(* Logix 5000 AddOnInstructionDefinition export; software revision 16.04 *)

ADD_ON_INSTRUCTION AOI_ICX35   (* revision 1.8 *)
// Add-On Instruction for ICX35 Industrial Cellular Gateway
// Revision note:
// 1.8    2018/06/14.
// This Revision is compatible with ICX35 firmware version 1.4 and later.
VAR_IN_OUT
   ICX35 : ICX35_ModuleDef; {required}
   ICX35_MSG_GET_STATUS : MESSAGE; {required}
   ICX35_MSG_READ_SMS : MESSAGE; {required}
   ICX35_MSG_RESET_STATUS : MESSAGE; {required}
   ICX35_MSG_WRITE_SMS : MESSAGE; {required}
   ICX35_MSG_CLEAR_SMS : MESSAGE; {required}
   ICX35_MSG_REBOOT : MESSAGE; {required}
END_VAR

ROUTINE Logic   (* ladder *)
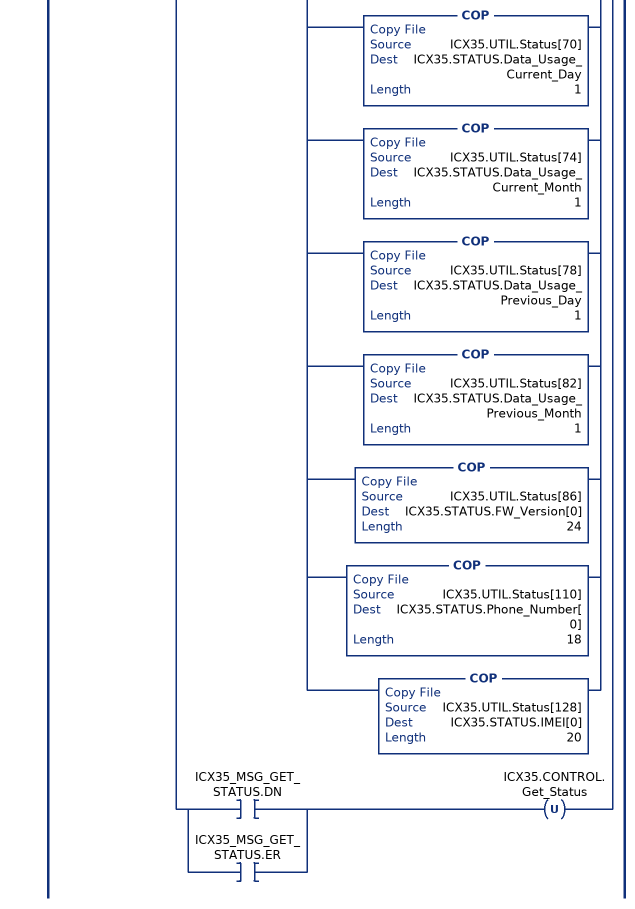
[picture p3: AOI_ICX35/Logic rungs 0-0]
   0: XIC(ICX35.CONTROL.Get_Status)[MSG(ICX35_MSG_GET_STATUS) ,XIC(ICX35_MSG_GET_STATUS.DN) [COP(ICX35.UTIL.Status[0],ICX35.STATUS.RSSI,4) ,COP(ICX35.UTIL.Status[4],ICX35.STATUS.MAC_Address[0],6) ,MVM(0,65280,ICX35.STATUS.WAN_IP[0]) ,MVM(ICX35.UTIL.Status[10],255,ICX35.STATUS.WAN_IP[0]) ,MVM(0,65280,ICX35.STATUS.WAN_IP[1]) ,MVM(ICX35.UTIL.Status[11],255,ICX35.STATUS.WAN_IP[1]) ,MVM(0,65280,ICX35.STATUS.WAN_IP[2]) ,MVM(ICX35.UTIL.Status[12],255,ICX35.STATUS.WAN_IP[2]) ,MVM(0,65280,ICX35.STATUS.WAN_IP[3]) ,MVM(ICX35.UTIL.Status[13],255,ICX35.STATUS.WAN_IP[3]) ,COP(ICX35.UTIL.Status[14],ICX35.STATUS.Cell_Net_Disconnects,1) ,COP(ICX35.UTIL.Status[18],ICX35.STATUS.LAN_KBytes_Sent,1) ,COP(ICX35.UTIL.Status[22],ICX35.STATUS.LAN_KBytes_Received,1) ,COP(ICX35.UTIL.Status[26],ICX35.STATUS.WAN_KBytes_Sent,1) ,COP(ICX35.UTIL.Status[30],ICX35.STATUS.WAN_KBytes_Received,1) ,COP(ICX35.UTIL.Status[34],ICX35.STATUS.SMS_MSGs_Sent,1) ,COP(ICX35.UTIL.Status[38],ICX35.STATUS.SMS_MSGs_Received,1) ,COP(ICX35.UTIL.Status[42],ICX35.STATUS.SMS_MSGs_Rx_Free_Buffer_Counter,1) ,COP(ICX35.UTIL.Status[46],ICX35.STATUS.PowerOnTime_Year,1) ,COP(ICX35.UTIL.Status[48],ICX35.STATUS.PowerOnTime_Month,1) ,COP(ICX35.UTIL.Status[50],ICX35.STATUS.PowerOnTime_Day,1) ,COP(ICX35.UTIL.Status[52],ICX35.STATUS.PowerOnTime_Hour,1) ,COP(ICX35.UTIL.Status[54],ICX35.STATUS.PowerOnTime_Minute,1) ,COP(ICX35.UTIL.Status[56],ICX35.STATUS.PowerOnTime_Second,1) ,COP(ICX35.UTIL.Status[58],ICX35.STATUS.Link_Time_Days,1) ,COP(ICX35.UTIL.Status[62],ICX35.STATUS.Link_Time_Hours,1) ,COP(ICX35.UTIL.Status[66],ICX35.STATUS.Link_Time_Minutes,1) ,COP(ICX35.UTIL.Status[68],ICX35.STATUS.Link_Time_Seconds,1) ,COP(ICX35.UTIL.Status[70],ICX35.STATUS.Data_Usage_Current_Day,1) ,COP(ICX35.UTIL.Status[74],ICX35.STATUS.Data_Usage_Current_Month,1) ,COP(ICX35.UTIL.Status[78],ICX35.STATUS.Data_Usage_Previous_Day,1) ,COP(ICX35.UTIL.Status[82],ICX35.STATUS.Data_Usage_Previous_Month,1) ,COP(ICX35.UTIL.Status[86],ICX35.STATUS.FW_Version[0],24) ,COP(ICX35.UTIL.Status[110],ICX35.STATUS.Phone_Number[0],18) ,COP(ICX35.UTIL.Status[128],ICX35.STATUS.IMEI[0],20) ] ,[XIC(ICX35_MSG_GET_STATUS.DN) ,XIC(ICX35_MSG_GET_STATUS.ER) ] OTU(ICX35.CONTROL.Get_Status) ];
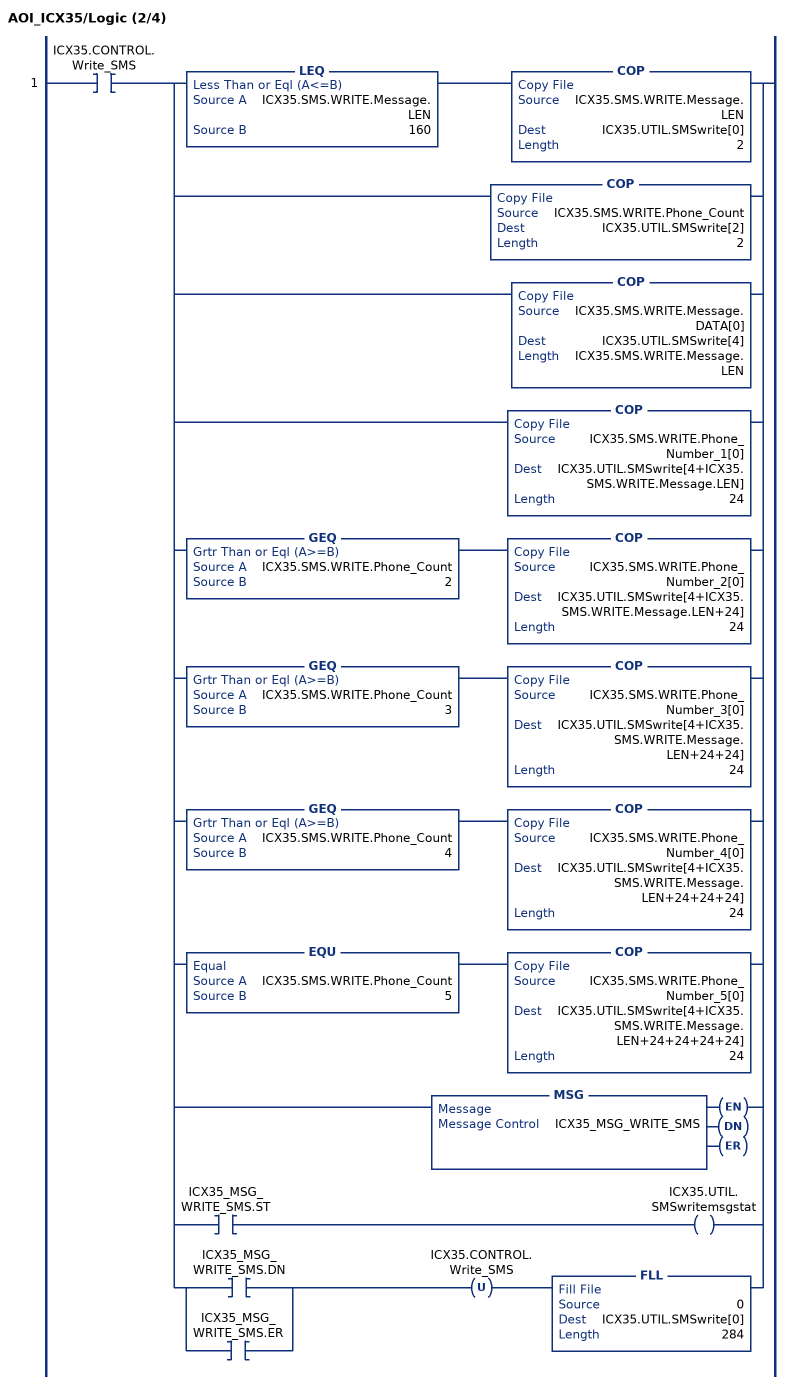
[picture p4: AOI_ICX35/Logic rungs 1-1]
   1: XIC(ICX35.CONTROL.Write_SMS)[LEQ(ICX35.SMS.WRITE.Message.LEN,160) COP(ICX35.SMS.WRITE.Message.LEN,ICX35.UTIL.SMSwrite[0],2) ,COP(ICX35.SMS.WRITE.Phone_Count,ICX35.UTIL.SMSwrite[2],2) ,COP(ICX35.SMS.WRITE.Message.DATA[0],ICX35.UTIL.SMSwrite[4],ICX35.SMS.WRITE.Message.LEN) ,COP(ICX35.SMS.WRITE.Phone_Number_1[0],ICX35.UTIL.SMSwrite[4+ICX35.SMS.WRITE.Message.LEN],24) ,GEQ(ICX35.SMS.WRITE.Phone_Count,2) COP(ICX35.SMS.WRITE.Phone_Number_2[0],ICX35.UTIL.SMSwrite[4+ICX35.SMS.WRITE.Message.LEN+24],24) ,GEQ(ICX35.SMS.WRITE.Phone_Count,3) COP(ICX35.SMS.WRITE.Phone_Number_3[0],ICX35.UTIL.SMSwrite[4+ICX35.SMS.WRITE.Message.LEN+24+24],24) ,GEQ(ICX35.SMS.WRITE.Phone_Count,4) COP(ICX35.SMS.WRITE.Phone_Number_4[0],ICX35.UTIL.SMSwrite[4+ICX35.SMS.WRITE.Message.LEN+24+24+24],24) ,EQU(ICX35.SMS.WRITE.Phone_Count,5) COP(ICX35.SMS.WRITE.Phone_Number_5[0],ICX35.UTIL.SMSwrite[4+ICX35.SMS.WRITE.Message.LEN+24+24+24+24],24) ,MSG(ICX35_MSG_WRITE_SMS) ,XIC(ICX35_MSG_WRITE_SMS.ST) OTE(ICX35.UTIL.SMSwritemsgstat) ,[XIC(ICX35_MSG_WRITE_SMS.DN) ,XIC(ICX35_MSG_WRITE_SMS.ER) ] OTU(ICX35.CONTROL.Write_SMS) FLL(0,ICX35.UTIL.SMSwrite[0],284) ];
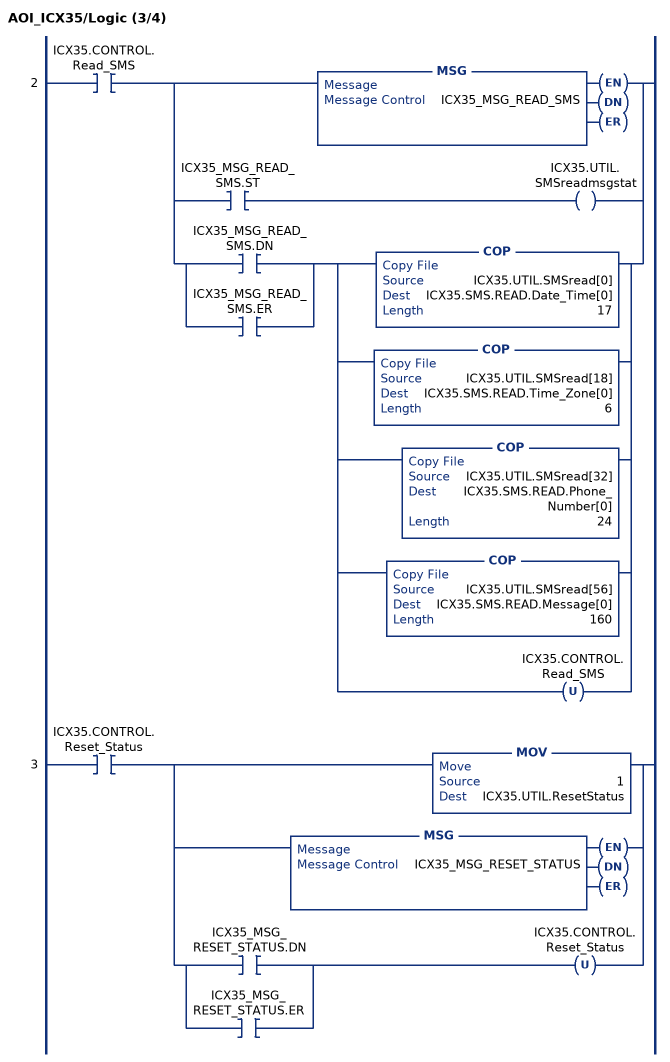
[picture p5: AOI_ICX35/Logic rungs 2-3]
   2: XIC(ICX35.CONTROL.Read_SMS)[MSG(ICX35_MSG_READ_SMS) ,XIC(ICX35_MSG_READ_SMS.ST) OTE(ICX35.UTIL.SMSreadmsgstat) ,[XIC(ICX35_MSG_READ_SMS.DN) ,XIC(ICX35_MSG_READ_SMS.ER) ] [COP(ICX35.UTIL.SMSread[0],ICX35.SMS.READ.Date_Time[0],17) ,COP(ICX35.UTIL.SMSread[18],ICX35.SMS.READ.Time_Zone[0],6) ,COP(ICX35.UTIL.SMSread[32],ICX35.SMS.READ.Phone_Number[0],24) ,COP(ICX35.UTIL.SMSread[56],ICX35.SMS.READ.Message[0],160) ,OTU(ICX35.CONTROL.Read_SMS) ] ];
   3: XIC(ICX35.CONTROL.Reset_Status)[MOV(1,ICX35.UTIL.ResetStatus) ,MSG(ICX35_MSG_RESET_STATUS) ,[XIC(ICX35_MSG_RESET_STATUS.DN) ,XIC(ICX35_MSG_RESET_STATUS.ER) ] OTU(ICX35.CONTROL.Reset_Status) ];
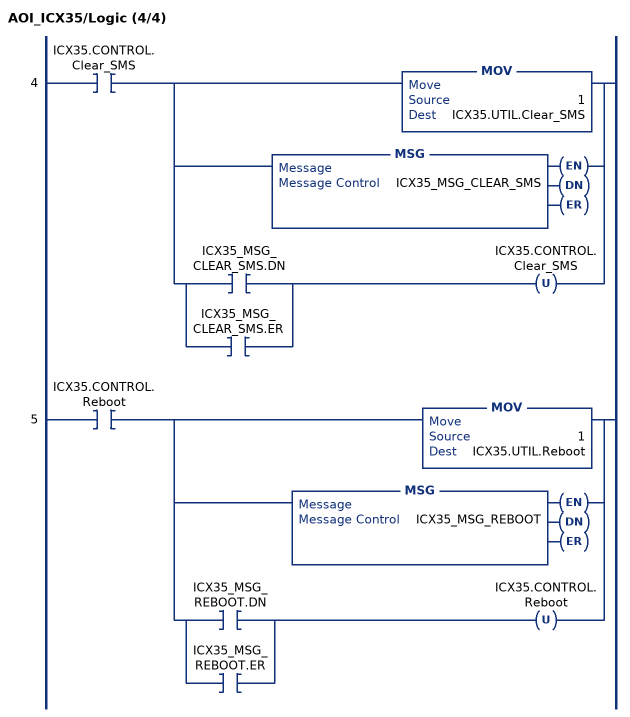
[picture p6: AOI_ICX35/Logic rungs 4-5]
   4: XIC(ICX35.CONTROL.Clear_SMS)[MOV(1,ICX35.UTIL.Clear_SMS) ,MSG(ICX35_MSG_CLEAR_SMS) ,[XIC(ICX35_MSG_CLEAR_SMS.DN) ,XIC(ICX35_MSG_CLEAR_SMS.ER) ] OTU(ICX35.CONTROL.Clear_SMS) ];
   5: XIC(ICX35.CONTROL.Reboot)[MOV(1,ICX35.UTIL.Reboot) ,MSG(ICX35_MSG_REBOOT) ,[XIC(ICX35_MSG_REBOOT.DN) ,XIC(ICX35_MSG_REBOOT.ER) ] OTU(ICX35.CONTROL.Reboot) ];
END_ROUTINE
END_ADD_ON_INSTRUCTION
